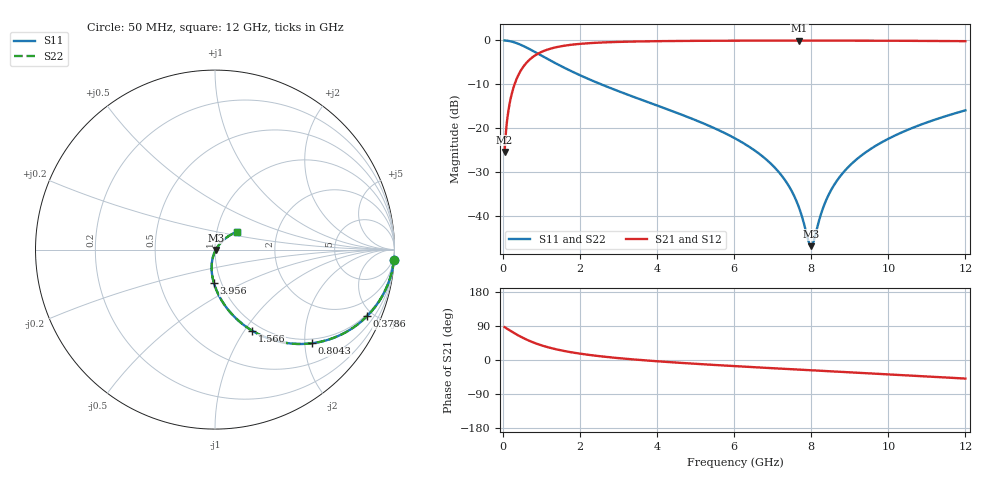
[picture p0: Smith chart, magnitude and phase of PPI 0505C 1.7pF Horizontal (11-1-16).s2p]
# MHz S MA R 50
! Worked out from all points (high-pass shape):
!   1601 points, 50 MHz to 12 GHz, reference 50 ohm
!   highest |S21| = -0.04 dB at 7.691 GHz (marker M1); lowest = -25.3 dB at 50 MHz (marker M2)
!   |S21| within 3 dB of the highest: 910.5 MHz to end of sweep
!   lowest |S11| = -46.8 dB at 7.997 GHz (marker M3), VSWR 1.01, Z = 50.4 - j0.219 ohm
!   |S11| at or under -10 dB: 2.556 GHz to end of sweep
!   |S22| runs from -46.8 to 0.0 dB; largest |S21 - S12| = 0
!   S11 on the Smith chart (normalised r, x): 50 MHz: 1, -35; 378.6 MHz: 0.90, -4.61; 804.3 MHz: 0.90, -2.16; 1.566 GHz: 0.90, -1.08; 3.956 GHz: 0.92, -0.35; 12 GHz: 1.26, +0.26
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50  0.9985 -3.3  0.05403 86.7  0.05403 86.7  0.9985 -3.3
191.9062  0.979 -12.4  0.2034 77.6  0.2034 77.6  0.979 -12.4
378.625  0.9249 -23.6  0.3795 66.3  0.3795 66.3  0.9249 -23.6
565.3438  0.8518 -33.5  0.5229 56.5  0.5229 56.5  0.8518 -33.5
804.3438  0.7513 -44.0  0.6587 45.9  0.6587 45.9  0.7513 -44.0
1162.844  0.6155 -55.9  0.7864 34.0  0.7864 34.0  0.6155 -55.9
1566.156  0.4968 -65.4  0.8658 24.4  0.8658 24.4  0.4968 -65.4
2044.156  0.3946 -73.5  0.9164 16.2  0.9164 16.2  0.3946 -73.5
3956.156  0.1851 -92.0  0.9793 -3.0  0.9793 -3.0  0.1851 -92.0
4038.312  0.1796 -92.6  0.9803 -3.6  0.9803 -3.6  0.1796 -92.6
6025  0.07692 -103.3  0.9928 -16.2  0.9928 -16.2  0.07692 -103.3
7085.562  0.03466 -105.1  0.9947 -22.2  0.9947 -22.2  0.03466 -105.1
7436.594  0.02151 -102.4  0.9949 -24.1  0.9949 -24.1  0.02151 -102.4
7690.531  0.01236 -94.3  0.995 -25.5  0.995 -25.5  0.01236 -94.3
7929.531  0.00524 -56.6  0.995 -26.7  0.995 -26.7  0.00524 -56.6
7996.75  0.004571 -28.4  0.9949 -27.1  0.9949 -27.1  0.004571 -28.4
8019.156  0.004637 -18.2  0.9949 -27.2  0.9949 -27.2  0.004637 -18.2
8362.719  0.01432 41.7  0.9947 -29.1  0.9947 -29.1  0.01432 41.7
8706.281  0.02678 48.6  0.9943 -30.9  0.9943 -30.9  0.02678 48.6
9251.5  0.04717 50.0  0.9933 -33.9  0.9933 -33.9  0.04717 50.0
10013.31  0.07655 48.0  0.9911 -38.0  0.9911 -38.0  0.07655 48.0
12000  0.1602 38.7  0.98 -49.0  0.98 -49.0  0.1602 38.7
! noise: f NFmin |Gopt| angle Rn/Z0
50  0.0008959  0.954  1.75  0.004378
1372  0.005506  0.7549  6.265  0.004526
2701  0.008672  0.7021  10.47  0.005659
4031  0.01147  0.6711  14.73  0.0066
5360  0.01409  0.6507  18.95  0.007469
6682  0.01664  0.6372  23.09  0.008318
8012  0.0192  0.6288  27.16  0.009195
9341  0.02182  0.6246  31.14  0.01013
1.067e+04  0.02452  0.6238  35  0.01114
1.2e+04  0.02738  0.6261  38.76  0.01228
